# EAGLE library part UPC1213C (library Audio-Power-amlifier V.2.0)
AUDIO POWER AMPLIEFIER AT 9-VOLT POWER SUPPLY
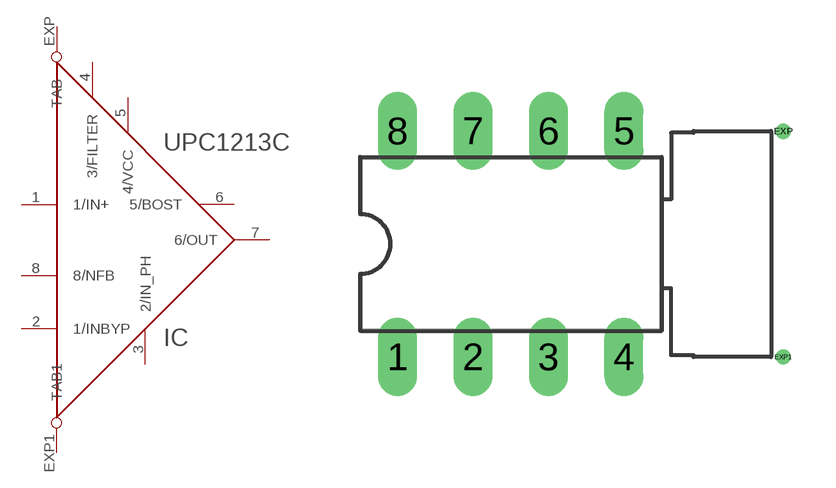
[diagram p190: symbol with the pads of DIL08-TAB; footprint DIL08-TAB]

Designator prefix IC

## UPC1213C  [DIL08-TAB]
1  1/IN+  in
2  1/INBYP  in
3  2/IN_PH  in
4  3/FILTER
5  4/VCC  pwr
6  5/BOST
7  6/OUT  out
8  8/NFB  in
EXP  TAB  pwr
EXP1  TAB1  pwr

## Footprint DIL08-TAB (pad centres in mm)
Dual In Line Package With TAB
drill 0.813 long: 1 -3.81,-3.81; 2 -1.27,-3.81; 3 1.27,-3.81; 4 3.81,-3.81; 5 3.81,3.81; 6 1.27,3.81; 7 -1.27,3.81; 8 -3.81,3.81
drill 0.01 pad 0.01: EXP 9.18,3.8; EXP1 9.18,-3.81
